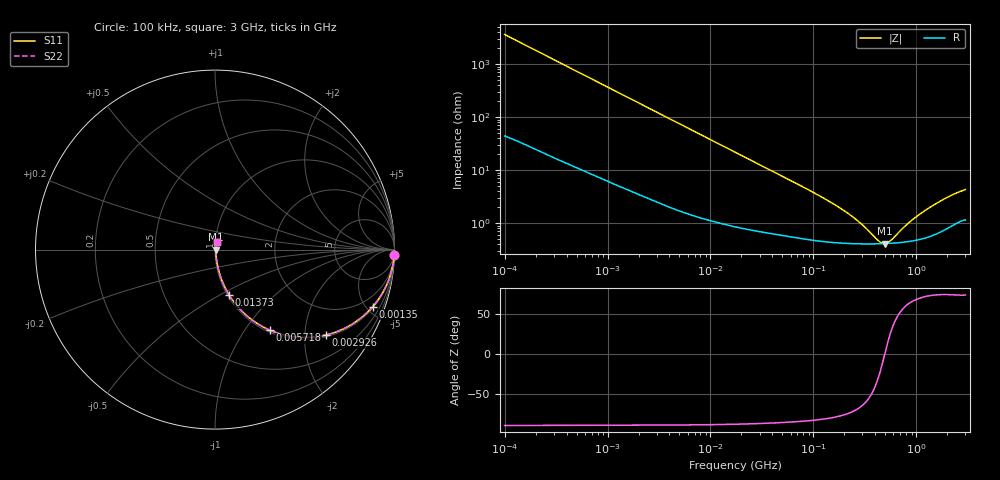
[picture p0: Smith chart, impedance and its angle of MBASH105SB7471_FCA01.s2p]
! MBASH105SB7471_FCA01  S-PARAMETER MODEL  ( Standard Model )
! Model Generated by TAIYO YUDEN Corporation (http://www.ty-top.com)
! Version 1.0
! TAIYO YUDEN Control No. 220601
! Copyright(c) 2019 TAIYO YUDEN CO.,LTD. All Rights Reserved.
! Product Description (link to TY-COMPAS)
! https://ds.yuden.co.jp/TYCOMPAS/or/detail?pn=MBASH105SB7471KFCA01&u=M
! Products Name : Multilayer Ceramic Capacitors
! Characteristics :
!  Capacitance : 470 [pF] , Rated Voltage : 100 [V] , TCC : X7R
!  Case Size : 1.0 x 0.5 / 0.039 x 0.02 [mm/inch] , Thickness : 0.5 / 0.02 [mm/inch]
!  (Conditions: Temperature = 25 [degC] , DC Bias Voltage = 0 [V])
! External Node Assignments :
!  1  o---| |---o  2
! GND o---------o GND
! Frequency Range : 100kHz  -  3GHz  [ 401 STEP ]
# MHZ S RI R 50
! Freq[MHz].  S11 Real  S11 Imag  S21 Real  S21 Imag  S12 Real  S12 Imag  S22 Real  S22 Imag
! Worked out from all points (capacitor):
!   401 points, 100 kHz to 3 GHz, reference 50 ohm
!   read as one part in series: C = 437 pF near 105.3 kHz
!   lowest |Z| = 414 mohm at 493.9 MHz (marker M1)
!   series resonance near 493.1 MHz, so ESL is about 240 pH
!   S11 on the Smith chart (normalised r, x): 100 kHz: 2, -73; 1.35 MHz: 1.10, -5.51; 2.926 MHz: 1.05, -2.56; 5.718 MHz: 1.03, -1.32; 13.73 MHz: 1.02, -0.55; 3 GHz: 1.02, +0.08
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0.1  0.9989 -0.0275  0.00109 0.0275  0.00109 0.0275  0.9989 -0.0275
0.259498  0.994 -0.0704  0.00596 0.0704  0.00596 0.0704  0.994 -0.0704
0.562235  0.9751 -0.1483  0.0249 0.1483  0.0249 0.1483  0.9751 -0.1483
1.350433  0.8793 -0.3172  0.1207 0.3172  0.1207 0.3172  0.8793 -0.3172
1.987766  0.775 -0.4083  0.225 0.4083  0.225 0.4083  0.775 -0.4083
2.925885  0.6194 -0.4756  0.3806 0.4756  0.3806 0.4756  0.6194 -0.4756
3.161081  0.5834 -0.4829  0.4166 0.4829  0.4166 0.4829  0.5834 -0.4829
5.718342  0.3078 -0.45  0.6922 0.45  0.6922 0.45  0.3078 -0.45
8.636841  0.1683 -0.3607  0.8317 0.3607  0.8317 0.3607  0.1683 -0.3607
13.7349  0.079 -0.253  0.921 0.253  0.921 0.253  0.079 -0.253
17.7727  0.0515 -0.2022  0.9485 0.2022  0.9485 0.2022  0.0515 -0.2022
37.52708  0.0166 -0.1002  0.9834 0.1002  0.9834 0.1002  0.0166 -0.1002
97.38194  0.00627 -0.0385  0.9937 0.0385  0.9937 0.0385  0.00627 -0.0385
216.4987  0.00436 -0.0147  0.9956 0.0147  0.9956 0.0147  0.00436 -0.0147
294.964  0.00415 -0.00862  0.9959 0.00862  0.9959 0.00862  0.00415 -0.00862
434.1712  0.00409 -0.00205  0.9959 0.00205  0.9959 0.00205  0.00409 -0.00205
493.8841  0.00412 2.69e-05  0.9959 -2.69e-05  0.9959 -2.69e-05  0.00412 2.69e-05
547.5153  0.00416 0.00169  0.9958 -0.00169  0.9958 -0.00169  0.00416 0.00169
848.5431  0.00459 0.00914  0.9954 -0.00914  0.9954 -0.00914  0.00459 0.00914
1186.261  0.00541 0.0159  0.9946 -0.0159  0.9946 -0.0159  0.00541 0.0159
1986.261  0.0087 0.0291  0.9913 -0.0291  0.9913 -0.0291  0.0087 0.0291
3000  0.0131 0.0406  0.9869 -0.0406  0.9869 -0.0406  0.0131 0.0406
